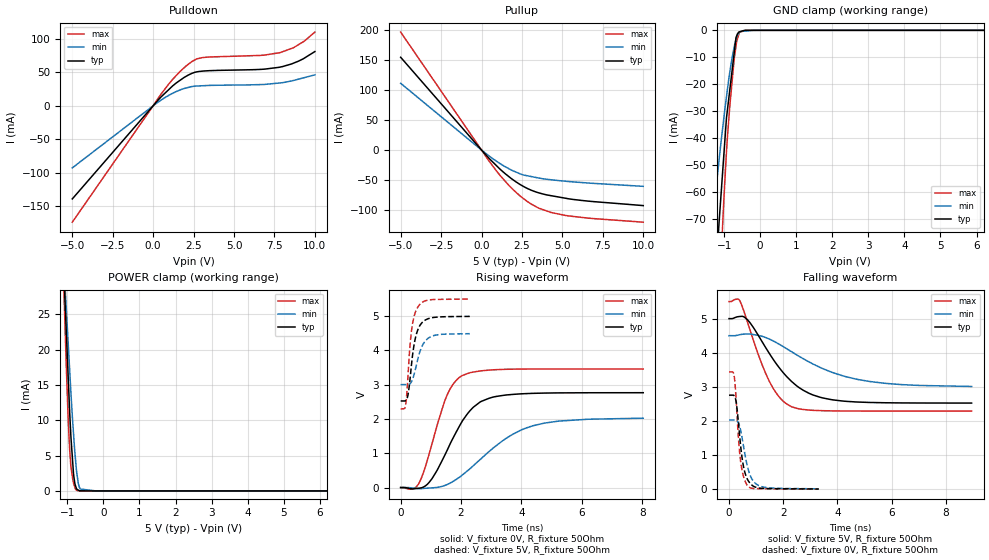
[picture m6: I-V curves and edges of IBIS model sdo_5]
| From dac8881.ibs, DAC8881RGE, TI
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|   sdo_5 Model
[Model]   sdo_5
Model_type   3-state
Polarity   Non-Inverting
Vmeas = 2.5
Vref = 2.5
Cref = 50pF
Rref = 50
|   typ   min   max
|   (nom PVT)   (fast PVT)   (slow PVT)
|C_comp from frequency sweep method (F=25MHz)
|C_comp   5.332e-12   4.452e-12   6.641e-12
|ON state : BUFFER OUTPUT TURNED HIGH
|C_comp   5.332e-12   4.452e-12   6.641e-12
|OFF state: BUFFER IN HIGH IMPEDANCE
|C_comp   3.357e-12   2.618e-12   4.089e-12
|C_comp from LC tank measurement(L=1nH)
|Resonant Frequency(Hz)   2.980e+09   3.260e+09   2.750e+09
C_comp   2.855e-12   2.386e-12   3.353e-12
|ON state : BUFFER OUTPUT TURNED HIGH
|Resonant Frequency(Hz)   2.980e+09   3.260e+09   2.750e+09
|C_comp   2.855e-12   2.386e-12   3.353e-12
|OFF state: BUFFER IN HIGH IMPEDANCE
|Resonant Frequency(Hz)   3.060e+09   3.380e+09   2.810e+09
|C_comp   2.708e-12   2.219e-12   3.211e-12
| Where nom  PVT is Nominal Process, 5V, 25C
|   Fast PVT is Strong Process,  5.5V, -40C
|   Slow PVT is Weak Process,   4.5V, 105C
[Voltage Range]   5   4.5   5.5
|Ambient Temperature   25   105   -40
|Junction Temperature
[Temperature Range]   25   105   -40
[Pullup Reference]   5   4.5   5.5
[Pulldown Reference]   0   0   0
[Power Clamp Reference]   5   4.5   5.5
[GND Clamp Reference]   0   0   0
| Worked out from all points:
|   slope of the pulldown table from 0 to 0.75 V, typ, clamps not added: 39 ohm
|   slope of the pullup table from 0 to 0.75 V, typ, clamps not added: 35 ohm
|   GND clamp passes 1 mA (typ) near -0.61 V on its own axis
|   POWER clamp passes 1 mA (typ) near -0.79 V on its own axis
|   falling waveform, V_fixture 5V, R_fixture 50Ohm: 20-80 % time 1.43ns typ, 2.31ns min, 950ps max; typ from 5 V to 2.52 V
|   rising waveform, V_fixture 0V, R_fixture 50Ohm: 20-80 % time 1.03ns typ, 1.76ns min, 728ps max; typ from 0 V to 2.77 V
|   rising waveform, V_fixture 5V, R_fixture 50Ohm: 20-80 % time 237ps typ, 305ps min, 192ps max; typ from 2.52 V to 4.99 V
|   falling waveform, V_fixture 0V, R_fixture 50Ohm: 20-80 % time 249ps typ, 324ps min, 199ps max; typ from 2.76 V to 0.006 V
[Pulldown]
|   Voltage   I(typ)   I(min)   I(max)
-5V       -138.8mA   -92.53mA   -173.4mA
500mV     13.49mA    8.631mA    17.73mA
1.221V    29.95mA    18.85mA    39.78mA
2.013V    43.58mA    26.38mA    58.84mA
2.376V    48.16mA    28.6mA     65.64mA
2.689V    50.54mA    29.43mA    69.9mA
3.08V     51.76mA    29.9mA     71.97mA
6.6V      54.2mA     31.6mA     75.05mA
7.854V    57.71mA    34.1mA     79.25mA
8.684V    63.6mA     37.8mA     86.61mA
9.345V    70.97mA    41.96mA    96.31mA
10V       80.82mA    46.08mA    109.8mA
[GND Clamp]
|   Voltage   I(typ)   I(min)   I(max)
-5V       -985.8mA   -691.1mA   -1.337A
-1.373V   -120.5mA   -78.44mA   -172.3mA
-1.228V   -89.79mA   -59.31mA   -127.7mA
-1.14V    -71.49mA   -48.28mA   -101.1mA
-1.083V   -60.78mA   -41.34mA   -84.28mA
-1.001V   -45.16mA   -31.88mA   -61.34mA
-935mV    -32.65mA   -24.79mA   -45.32mA
-841.5mV  -22.07mA   -15.45mA   -28.14mA
-726mV    -9.005mA   -6.593mA   -11.41mA
-670mV    -2.669mA   -3.337mA   -5.792mA
-558mV    -501.8uA   -444.4uA   -661.9uA
10V       0A         0A         0A
[Pullup]
|   Voltage   I(typ)   I(min)   I(max)
-5V       154.7mA    111.3mA    196.7mA
445.5mV   -13.25mA   -9.509mA   -17.57mA
1.155V    -32.17mA   -22.82mA   -42.6mA
1.672V    -43.93mA   -30.88mA   -58.38mA
2.376V    -57.35mA   -39.61mA   -76.37mA
3.08V     -67.1mA    -44.26mA   -90.21mA
3.52V     -71.26mA   -46.56mA   -96.68mA
4.301V    -76.14mA   -49.62mA   -104.2mA
5.192V    -80.41mA   -52.04mA   -109.1mA
6.6V      -85.22mA   -55.01mA   -113.6mA
10V       -92.7mA    -60.57mA   -120.4mA
[POWER Clamp]
|   Voltage   I(typ)   I(min)   I(max)
-5V       296.2mA    257.8mA    340.9mA
-1.095V   30.44mA    31.83mA    28.11mA
-1.089V   29.77mA    31.27mA    27.19mA
-1.028V   22.39mA    25.66mA    17.46mA
-979mV    16.36mA    21.07mA    10.45mA
-935mV    10.99mA    16.99mA    5.714mA
-896.5mV  7.301mA    13.46mA    3.237mA
-830mV    2.453mA    8.167mA    1.151mA
-742.5mV  271.2uA    2.657mA    80.03uA
-643.5mV  19.82uA    269.8uA    1.628uA
-202.5mV  0A         0A         512.7nA
10V       0A         0A         0A
[Ramp]
R_load = 50
|   typ   min   max
dV/dt_r   1.65905/1.03062e-09   1.2189/1.76718e-09   2.07302/7.27087e-10
dV/dt_f   1.48539/1.43128e-09   0.899291/2.34495e-09   1.92529/9.49842e-10
[Falling Waveform]
V_fixture = 5V
V_fixture_min = 4.5V
V_fixture_max = 5.5V
R_fixture = 50Ohm
|   Time   V(typ)   V(min)   V(max)
0s        5V         4.5V       5.5V
400ps     5.063V     4.53V      5.522V
770ps     4.885V     4.552V     4.68V
1.205ns   4.345V     4.485V     3.68V
1.475ns   3.996V     4.406V     3.183V
1.895ns   3.519V     4.23V      2.664V
2.31ns    3.157V     4.03V      2.418V
3.34ns    2.701V     3.577V     2.305V
4.765ns   2.555V     3.216V     2.291V
8.955ns   2.525V     3.012V     2.291V
[Rising Waveform]
V_fixture = 0V
V_fixture_min = 0V
V_fixture_max = 0V
R_fixture = 50Ohm
|   Time   V(typ)   V(min)   V(max)
0s        1.647nV    1.968nV    1.531nV
605ps     -20.15mV   -30.35mV   122.2mV
945ps     152.5mV    -13.8mV    983.5mV
1.475ns   967.6mV    65.06mV    2.561V
1.735ns   1.442V     178.2mV    3.011V
2.045ns   1.944V     368.4mV    3.267V
2.415ns   2.347V     643.9mV    3.369V
2.915ns   2.599V     1.041V     3.423V
4.365ns   2.746V     1.798V     3.456V
8.035ns   2.765V     2.022V     3.456V
[Rising Waveform]
V_fixture = 5V
V_fixture_min = 4.5V
V_fixture_max = 5.5V
R_fixture = 50Ohm
|   Time   V(typ)   V(min)   V(max)
0s        2.524V     3.001V     2.291V
160ps     2.529V     3.001V     2.383V
245ps     2.715V     3.002V     3.294V
300ps     3.078V     3.019V     4.034V
355ps     3.55V      3.078V     4.535V
450ps     4.19V      3.314V     5.007V
565ps     4.591V     3.735V     5.258V
760ps     4.849V     4.205V     5.423V
1.005ns   4.945V     4.402V     5.475V
2.29ns    4.99V      4.486V     5.495V
[Falling Waveform]
V_fixture = 0V
V_fixture_min = 0V
V_fixture_max = 0V
R_fixture = 50Ohm
|   Time   V(typ)   V(min)   V(max)
0s        2.756V     2.028V     3.44V
185ps     2.746V     2.028V     3.339V
270ps     2.52V      2.021V     2.525V
350ps     1.926V     1.947V     1.476V
420ps     1.337V     1.756V     868.6mV
530ps     684.8mV    1.284V     390.2mV
680ps     289.8mV    666mV      103.5mV
890ps     92.41mV    244.2mV    21.58mV
1.205ns   25.34mV    74.19mV    15.42mV
3.31ns    5.645mV    11.59mV    1.095mV
